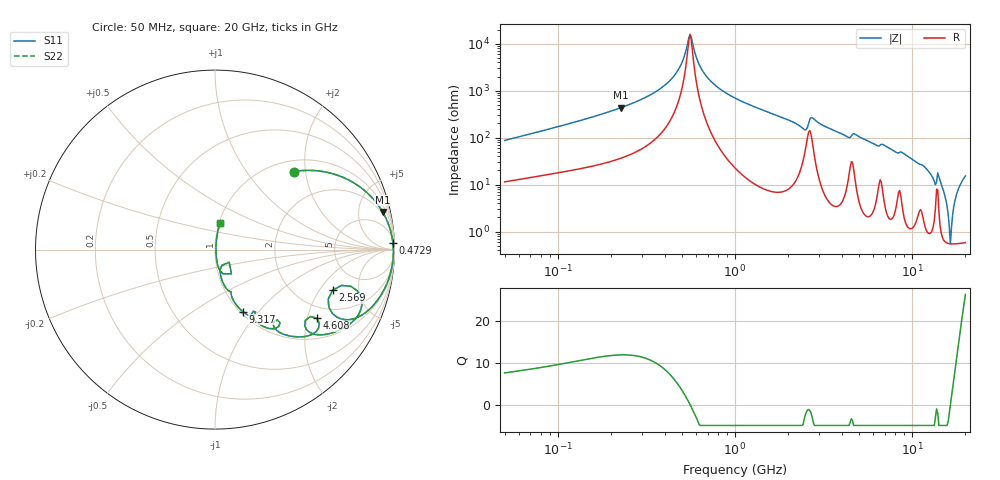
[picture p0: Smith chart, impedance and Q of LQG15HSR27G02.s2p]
!Murata Part Number: LQG15HSR27G02
!These Parameters are Measured in Series Mode Connection
!  o--[Z]--o
!Port1  Port2
!  o-------o
!Freq. Start=50[MHz] Stop=20[GHz], 401[Steps]
# Hz S RI R 50
!Freq.(Hz) S11(Real) S11(Imag) S21(Real) S21(Imag) S12(Real) S12(Imag) S22(Real) S22(Imag)
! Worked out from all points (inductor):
!   401 points, 50 MHz to 20 GHz, reference 50 ohm
!   read as one part in series: L = 269 nH near 51.52 MHz
!   highest Q = 11.9 at 227 MHz (marker M1), where L = 304 nH
!   self-resonance near 549.3 MHz
!   S11 on the Smith chart (normalised r, x): 50 MHz: 1.23, +1.73; 472.9 MHz: 11, +51; 2.569 GHz: 3.05, -2.66; 4.608 GHz: 1.60, -2.29; 9.317 GHz: 1.03, -0.83; 20 GHz: 1.01, +0.31
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5e7  0.4395 0.4347  0.5605 -0.4347  0.5605 -0.4347  0.4395 0.4347
1.364002e8  0.8262 0.3349  0.1738 -0.3349  0.1738 -0.3349  0.8262 0.3349
2.269813e8  0.9338 0.2101  0.0662 -0.2101  0.0662 -0.2101  0.9338 0.2101
3.721004e8  0.9816 0.0916  0.0184 -0.0916  0.0184 -0.0916  0.9816 0.0916
4.728708e8  0.9912 0.0371  0.00884 -0.0371  0.00884 -0.0371  0.9912 0.0371
5.575697e8  0.9937 -3.75e-06  0.00631 3.75e-06  0.00631 3.75e-06  0.9937 -3.75e-06
6.285508e8  0.9936 -0.0272  0.00644 0.0272  0.00644 0.0272  0.9936 -0.0272
6.87656e8  0.9924 -0.0479  0.00764 0.0479  0.00764 0.0479  0.9924 -0.0479
1e9  0.9755 -0.1393  0.0245 0.1393  0.0245 0.1393  0.9755 -0.1393
2.279204e9  0.7574 -0.3888  0.2426 0.3888  0.2426 0.3888  0.7574 -0.3888
2.569357e9  0.6554 -0.2266  0.3446 0.2266  0.3446 0.2266  0.6554 -0.2266
2.728004e9  0.8111 -0.2591  0.1889 0.2591  0.1889 0.2591  0.8111 -0.2591
3.572216e9  0.6765 -0.4558  0.3235 0.4558  0.3235 0.4558  0.6765 -0.4558
4.608136e9  0.5669 -0.3823  0.4331 0.3823  0.4331 0.3823  0.5669 -0.3823
7.442007e9  0.2662 -0.4265  0.7338 0.4265  0.7338 0.4265  0.2662 -0.4265
9.316812e9  0.1547 -0.3456  0.8453 0.3456  0.8453 0.3456  0.1547 -0.3456
1.438523e10  0.0272 -0.116  0.9728 0.116  0.9728 0.116  0.0272 -0.116
1.527346e10  0.00961 -0.0588  0.9904 0.0588  0.9904 0.0588  0.00961 -0.0588
1.597544e10  0.00608 -0.023  0.9939 0.023  0.9939 0.023  0.00608 -0.023
1.646126e10  0.00544 9.3e-05  0.9946 -9.3e-05  0.9946 -9.3e-05  0.00544 9.3e-05
1.800918e10  0.0102 0.0682  0.9898 -0.0682  0.9898 -0.0682  0.0102 0.0682
2e10  0.0281 0.1474  0.9719 -0.1474  0.9719 -0.1474  0.0281 0.1474
